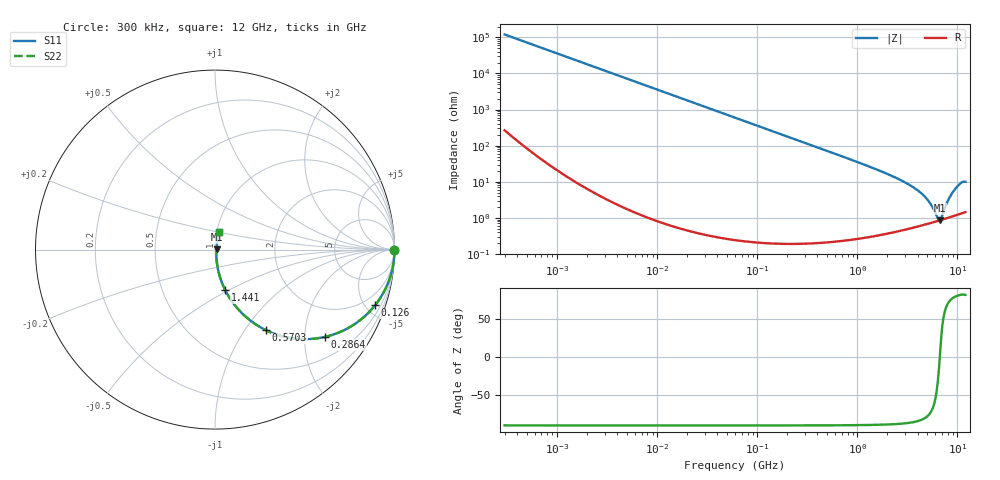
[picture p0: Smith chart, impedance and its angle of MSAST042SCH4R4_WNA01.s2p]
! MSAST042SCH4R4_WNA01  S-PARAMETER MODEL  ( General Type )
! Model Generated by TAIYO YUDEN Corporation (http://www.ty-top.com)
! Version 1.0
! TAIYO YUDEN Control No. 150820
! Copyright(c) 2015 TAIYO YUDEN CO.,LTD. All Rights Reserved.
! Product Description (link to TY-COMPAS)
! https://ds.yuden.co.jp/TYCOMPAS/or/detail?pn=MSAST042SCH4R4BWNA01&u=M
! Products Name : Multilayer Ceramic Capacitors
! Characteristics :
!  Capacitance : 4.4 pF , Rated Voltage : 25V , TCC : CH / C0H
!  Case Size : 0.4 x 0.2 / 0.016 x 0.008 [mm/inch] , Thickness : 0.2 / 0.008 [mm/inch]
!  (Conditions: Temperature = 25 degC , DC Bias Current/Voltage = 0A / 0V)
! External Node Assignments :
!  1  o---| |---o  2
! GND o---------o GND
! Frequency Range : 0.3MHz  -  12000MHz  [ 401 STEP ]
# MHz S RI R 50
! Freq[MHz].  S11 Real  S11 Imag  S21 Real  S21 Imag  S12 Real  S12 Imag  S22 Real  S22 Imag
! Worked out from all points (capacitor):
!   401 points, 300 kHz to 12 GHz, reference 50 ohm
!   read as one part in series: C = 4.4 pF near 316.3 kHz
!   lowest |Z| = 862 mohm at 6.7 GHz (marker M1)
!   series resonance near 6.664 GHz, so ESL is about 130 pH
!   S11 on the Smith chart (normalised r, x): 300 kHz: open; 126 MHz: 1.00, -5.74; 286.4 MHz: 1.00, -2.52; 570.3 MHz: 1.00, -1.26; 1.441 GHz: 1.01, -0.48; 12 GHz: 1.03, +0.20
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0.3  1 -0.00083  2.53e-06 0.00083  2.53e-06 0.00083  1 -0.00083
1.769972  1 -0.0049  2.58e-05 0.0049  2.58e-05 0.0049  1 -0.0049
10.44266  0.9992 -0.0289  0.00084 0.0289  0.00084 0.0289  0.9992 -0.0289
60  0.9731 -0.1615  0.0269 0.1615  0.0269 0.1615  0.9731 -0.1615
125.9782  0.8915 -0.3107  0.1085 0.3107  0.1085 0.3107  0.8915 -0.3107
187.4445  0.7876 -0.4085  0.2124 0.4085  0.2124 0.4085  0.7876 -0.4085
286.3882  0.6134 -0.4862  0.3866 0.4862  0.3866 0.4862  0.6134 -0.4862
353.9943  0.5091 -0.499  0.4909 0.499  0.4909 0.499  0.5091 -0.499
570.2811  0.2844 -0.4494  0.7156 0.4494  0.7156 0.4494  0.2844 -0.4494
894.6982  0.1376 -0.3414  0.8624 0.3414  0.8624 0.3414  0.1376 -0.3414
1441.349  0.0567 -0.2249  0.9433 0.2249  0.9433 0.2249  0.0567 -0.2249
2088.533  0.0273 -0.1513  0.9727 0.1513  0.9727 0.1513  0.0273 -0.1513
3190.978  0.0124 -0.0859  0.9876 0.0859  0.9876 0.0859  0.0124 -0.0859
4270.516  0.00845 -0.0493  0.9916 0.0493  0.9916 0.0493  0.00845 -0.0493
5140.631  0.0077 -0.0282  0.9923 0.0282  0.9923 0.0282  0.0077 -0.0282
6354.153  0.00819 -0.00526  0.9918 0.00526  0.9918 0.00526  0.00819 -0.00526
6699.894  0.00852 0.000637  0.9915 -0.000637  0.9915 -0.000637  0.00852 0.000637
7064.448  0.00897 0.00783  0.991 -0.00783  0.991 -0.00783  0.00897 0.00783
8064.993  0.0108 0.0285  0.9892 -0.0285  0.9892 -0.0285  0.0108 0.0285
8966.534  0.0134 0.0489  0.9866 -0.0489  0.9866 -0.0489  0.0134 0.0489
10511.28  0.0196 0.0826  0.9804 -0.0826  0.9804 -0.0826  0.0196 0.0826
12000  0.0236 0.0954  0.9764 -0.0954  0.9764 -0.0954  0.0236 0.0954
